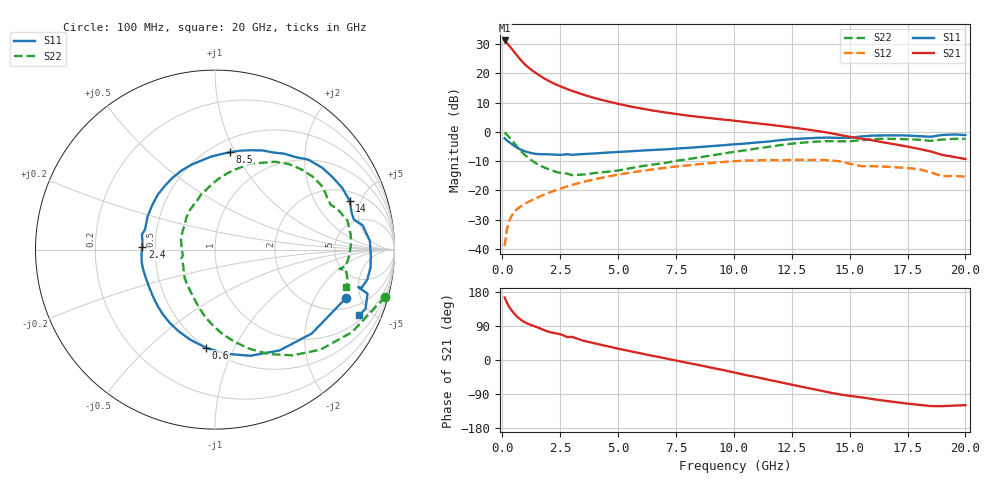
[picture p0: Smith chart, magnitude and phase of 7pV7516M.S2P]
! Infineon Technologies  Discrete & RF Semiconductors
! bfp620
! VCE = 0.75 V,  IC =  16 mA
! Common Emitter S-Parameters:  Sep 2002
# GHz  S  MA  R  50
!  f  S11  S21  S12  S22
! GHz  MAG  ANG  MAG  ANG  MAG  ANG  MAG  ANG
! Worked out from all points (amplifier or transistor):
!   59 points, 100 MHz to 20 GHz, reference 50 ohm
!   highest |S21| = 31.2 dB at 100 MHz (marker M1)
!   |S21| within 3 dB of that: start of sweep to 425 MHz
!   unconditionally stable (mu >= 1): 3.636 GHz to 10.28 GHz; 17.02 GHz to end of sweep
!   at 1 GHz: K = 0.64, MSG = 23.6 dB, |S12| = -24.4 dB
!   at 5.5 GHz: K = 1.04, MAG = 10.1 dB, |S12| = -14.0 dB
!   at 20 GHz: K = 1.47, MAG = -1.1 dB, |S12| = -15.3 dB
!   S11 on the Smith chart (normalised r, x): 100 MHz: 2.69, -3.68; 600 MHz: 0.50, -0.78; 2.4 GHz: 0.42, +0.02; 8.5 GHz: 0.62, +0.96; 14 GHz: 2.67, +3.99; 20 GHz: 1.29, -4.27
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0.1  0.7773 -20.4  36.28 165.1  0.0112 82.8  0.9842 -15.5
0.2  0.7137 -40.9  32.64 151.2  0.022 70.8  0.8911 -31.1
0.3  0.6671 -57.4  29.46 140.1  0.0302 64.6  0.8098 -43.5
0.4  0.6237 -71.5  26.43 131.1  0.0366 60.0  0.7303 -53.8
0.5  0.5834 -84.1  23.57 123.5  0.0418 56.5  0.654 -62.8
0.6  0.5486 -95.4  20.99 116.8  0.0463 53.8  0.5845 -70.9
0.7  0.52 -105.6  18.73 111.1  0.0501 51.8  0.5238 -78.2
0.8  0.4972 -114.4  16.81 106.2  0.0536 50.3  0.4726 -84.8
0.9  0.4786 -122.1  15.22 102.1  0.0569 49.3  0.4301 -90.6
1.1  0.4502 -134.5  12.81 95.8  0.063 48.2  0.3656 -100.2
1.4  0.4241 -148.6  10.42 88.9  0.0721 47.3  0.301 -112.0
1.8  0.415 -164.5  8.227 79.1  0.0847 45.8  0.2481 -128.9
2.4  0.4058 177.9  6.236 69.4  0.104 42.9  0.2032 -149.7
3.5  0.4183 153.9  4.31 50.9  0.1401 34.9  0.1867 176.7
5  0.4529 127.7  3.008 29.9  0.1864 21.7  0.2185 140.3
7  0.5017 98.7  2.152 5.0  0.2426 2.9  0.2931 109.2
8.5  0.5496 81.1  1.801 -13.5  0.281 -12.6  0.3657 92.6
10.5  0.631 59.0  1.473 -39.5  0.3234 -36.0  0.4848 71.8
13.5  0.788 25.8  1.05 -77.7  0.3312 -70.7  0.6791 36.8
14  0.7982 19.9  0.979 -84.1  0.3303 -77.4  0.6949 30.1
17  0.8725 -6.5  0.609 -111.3  0.2487 -101.5  0.7568 1.2
20  0.8833 -24.3  0.344 -119.2  0.1719 -112.8  0.7606 -15.9
